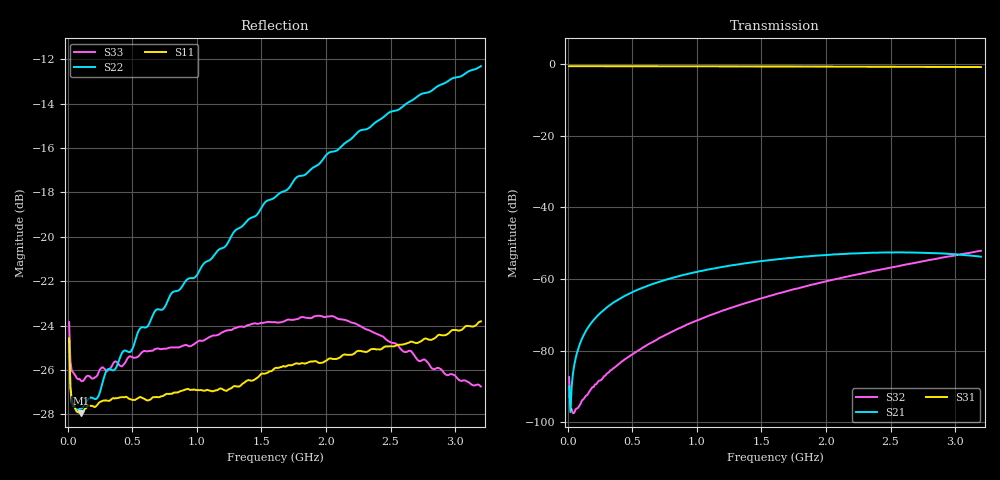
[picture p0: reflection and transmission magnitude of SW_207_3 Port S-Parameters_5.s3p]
! Created _Nov-02-2022_09-58-32
! Type : General
! Retest Level : 0
! Program : FASTESt Rev. 859
! DUT_TempC = 25.0
! Set_V1_Supply_V = 0.0
! V1_Supply_V = -0.0001
! V1_Supply_I = -5e-06
! Set_V2_Supply_V = 3.0
! V2_Supply_V = 3.0007
! V2_Supply_I = -6e-06
! RunID = 5
! SN = 3
! Comment = SW-207_SB3_RFc-RF2_room
! Input_Power = 5.0
! Measurement_Comment = None
! Freq	S11db	S11deg	S12db	S12deg	S13db	S13deg	S21db	S21deg	S22db	S22deg	S23db	S23deg	S31db	S31deg	S32db	S32deg	S33db	S33deg
# Hz S dB R 50
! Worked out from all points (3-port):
!   320 points, 10 MHz to 3.2 GHz, reference 50 ohm
!   strongest paths, dB at 10 MHz, 810 MHz, 1.61 GHz, 2.41 GHz, 3.2 GHz:
!     S31: -0.6, -0.6, -0.7, -0.7, -0.8
!     S21: -90.0, -59.7, -54.5, -52.6, -53.7
!     S32: -87.3, -74.6, -64.2, -57.4, -52.1
!   lowest |S11| = -28.0 dB at 100 MHz (marker M1), VSWR 1.08, Z = 54 - j1.21 ohm
!   |S11| at or under -10 dB: start of sweep to end of sweep
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1e7  -24.58 -43.7  -89.84 -123.0  -0.58 1.2
     -90.02 -123.4  -24.65 -40.5  -87.38 -112.5
     -0.58 1.2  -87.34 -113.3  -23.85 -40.4
1e8  -27.96 -16.3  -77.47 78.2  -0.59 -8.7
     -77.41 78.4  -27.75 -3.6  -94.61 -101.8
     -0.59 -8.7  -94.71 -102.6  -26.48 -14.6
3.6e8  -27.29 -30.9  -66.40 58.5  -0.60 -31.4
       -66.40 58.5  -26.00 -0.6  -84.64 -157.4
       -0.60 -31.4  -84.73 -158.4  -25.64 -30.4
8.8e8  -26.94 -91.5  -58.97 17.0  -0.63 -76.3
       -58.97 16.7  -22.29 -25.2  -73.39 139.4
       -0.62 -76.3  -73.44 139.2  -24.94 -86.2
1.23e9  -26.95 -135.3  -56.40 -11.1  -0.65 -106.4
        -56.42 -11.4  -20.36 -52.2  -68.42 105.9
        -0.65 -106.4  -68.44 105.7  -24.23 -123.8
1.61e9  -25.91 177.0  -54.53 -41.9  -0.68 -139.0
        -54.51 -41.9  -18.20 -81.7  -64.16 74.2
        -0.67 -139.0  -64.18 74.2  -23.85 -165.9
1.98e9  -25.66 133.8  -53.32 -72.3  -0.71 -170.7
        -53.34 -72.4  -16.48 -113.4  -60.78 45.0
        -0.70 -170.7  -60.80 44.9  -23.61 158.6
2.33e9  -25.14 99.1  -52.70 -101.1  -0.74 159.3
        -52.68 -101.2  -15.11 -141.9  -58.03 18.4
        -0.74 159.3  -58.01 18.1  -24.21 124.6
2.79e9  -24.63 56.8  -52.71 -138.8  -0.78 119.8
        -52.68 -138.9  -13.50 179.4  -54.73 -15.3
        -0.78 119.8  -54.73 -15.4  -25.68 77.7
3.2e9  -23.81 18.5  -53.78 -171.8  -0.83 84.5
       -53.73 -172.1  -12.31 144.3  -52.08 -44.4
       -0.82 84.4  -52.08 -44.6  -26.75 27.0
